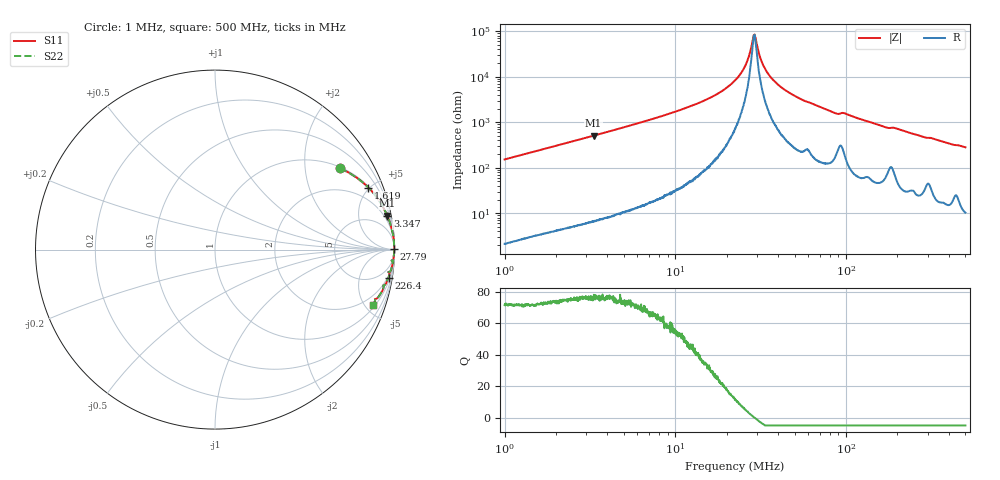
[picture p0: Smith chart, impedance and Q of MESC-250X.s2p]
!s-Parameter Generated by FASTRON Sdn. Bhd.
!FASTRON P/N : MESC-250X
!Keysight Technologies,E4991B,MY54100416,A.01.15
!Date: Fri Mar 27 09:24:28 2026
!Version  : Rev00 Fri Mar 27 09:24:28 2026
!Data & Calibration Information:
!PortZ  Port1:50+j0  Port2:50+j0
!When reading, reference impedance value at option line is always used.
!Remarks : This data is being provided solely for informational purposes.
!Freq	S11	S21	S12	S22
# Hz S dB R 50
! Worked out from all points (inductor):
!   1601 points, 1 MHz to 500 MHz, reference 50 ohm
!   read as one part in series: L = 24.2 uH near 1.032 MHz
!   highest Q = 76.7 at 3.321 MHz (marker M1), where L = 24.3 uH
!   self-resonance near 29.01 MHz
!   S11 on the Smith chart (normalised r, x): 1 MHz: 1.04, +3.05; 1.619 MHz: 1.07, +4.92; 3.347 MHz: 1, +10; 27.79 MHz: open; 226.4 MHz: 2, -12; 500 MHz: 1.21, -5.62
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1000000  -1.61 33.0  -5.28 -56.2  -5.28 -56.2  -1.61 33.0
1618714  -0.70 22.0  -8.53 -67.2  -8.53 -67.2  -0.70 22.0
2820919  -0.25 13.1  -12.92 -76.2  -12.92 -76.2  -0.25 13.1
3320768  -0.19 11.1  -14.29 -78.1  -14.29 -78.1  -0.19 11.1
3346665  -0.18 11.0  -14.36 -78.2  -14.36 -78.2  -0.18 11.0
7957584  -0.04 4.4  -22.27 -84.7  -22.27 -84.7  -0.04 4.4
1.540092e7  -0.01 1.8  -30.17 -86.4  -30.17 -86.4  -0.01 1.8
2.236068e7  -0.01 0.7  -38.34 -84.2  -38.34 -84.2  -0.01 0.7
2.55175e7  -0.01 0.3  -44.39 -79.3  -44.39 -79.3  -0.01 0.3
2.779387e7  -0.01 0.1  -52.78 -59.0  -52.78 -59.0  -0.01 0.1
2.867106e7  -0.01 0.0  -57.77 -25.5  -57.77 -25.5  -0.01 0.0
2.934708e7  -0.01 -0.0  -57.57 22.0  -57.57 22.0  -0.01 -0.0
3.147229e7  -0.01 -0.2  -48.23 71.6  -48.23 71.6  -0.01 -0.2
3.310225e7  -0.01 -0.3  -44.24 77.3  -44.24 77.3  -0.01 -0.3
3.911941e7  -0.01 -0.8  -37.16 83.1  -37.16 83.1  -0.01 -0.8
4.843613e7  -0.02 -1.4  -32.21 84.4  -32.21 84.4  -0.02 -1.4
6.307767e7  -0.03 -2.2  -28.26 83.7  -28.26 83.7  -0.03 -2.2
8.673569e7  -0.08 -3.6  -24.02 79.9  -24.02 79.9  -0.08 -3.6
9.783413e7  -0.08 -3.6  -24.04 79.4  -24.04 79.4  -0.08 -3.6
1.77937e8  -0.21 -7.5  -17.68 75.8  -17.68 75.8  -0.21 -7.5
2.263869e8  -0.18 -9.2  -15.90 78.0  -15.90 78.0  -0.18 -9.2
5e8  -0.62 -19.3  -9.60 68.6  -9.60 68.6  -0.62 -19.3
